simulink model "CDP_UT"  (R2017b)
settings: Solver=FixedStepDiscrete  StartTime=0.0  StopTime=10.0  FixedStep=0.01  RelTol=1e-3  EnableMultiTasking=on
undefined symbols (not defined in the file): ASWTYPE_FALSE, ASWTYPE_TRUE, CaCDP_CellTempNTCVoltTable_mV, CaCDP_CellTempTable_C, CaCDP_CMUPCBTempNTCVoltTable_mV, CaCDP_CMUPCBTempTable_C, CbCDP_DiffBusbarTempStateCheck_flg, CbCDP_DiffCellTempStateCheck_flg, CbCDP_DiffCellVoltStateCheck_flg, CbCDP_IgnorUpdateVld_flg, CbCDP_MaxBusbarTempStateCheck_flg, CbCDP_MaxCellTempStateCheck_flg, CbCDP_MaxCellVoltStateCheck_flg, CbCDP_MinBusbarTempStateCheck_flg, CbCDP_MinCellTempStateCheck_flg, CbCDP_MinCellVoltStateCheck_flg, CcCDP_AFETempConfig_numb, CcCDP_AFETempFltThd_C, CcCDP_AFETempFltThdHys_C, CcCDP_BusbarTempRngFltHiThrd_C, CcCDP_BusbarTempRngFltLowThrd_C, CcCDP_CellDiffFltLevel1_mV, CcCDP_CellDiffFltLevel2_mV, CcCDP_CellDiffFltLevel3_mV, CcCDP_CellTempLowerLimit_C, CcCDP_CellTempRngFltHiThrd_C, CcCDP_CellTempRngFltLowThrd_C, CcCDP_CellTempUpperLimit_C, CcCDP_CellVoltConfig_numb, CcCDP_CellVoltLowerLimit_mV, CcCDP_CellVoltRngHiThrd_mV, CcCDP_CellVoltRngLowThrd_mV, CcCDP_CellVoltUpdateThrd_numb, CcCDP_CellVoltUpperLimit_mV, CcCDP_ChrgMaxCellTempFltLv1Thrd_C, CcCDP_ChrgMaxCellTempFltLv2Thrd_C, CcCDP_ChrgMaxCellTempFltLv3Thrd_C, CcCDP_ChrgMaxCellTempReturnDiff_C, CcCDP_ChrgMinCellTempFltLv1Thrd_C, CcCDP_ChrgMinCellTempFltLv2Thrd_C, CcCDP_ChrgMinCellTempFltLv3Thrd_C, CcCDP_ChrgMinCellTempReturnDiff_C, CcCDP_CMUPCBTempConfig_numb, CcCDP_CMUPCBTempFltThd_C, CcCDP_CMUPCBTempFltThdHys_C, CcCDP_DiffBusbarTempFltLevel1Thrd_C, CcCDP_DiffBusbarTempFltLevel2Thrd_C, CcCDP_DiffBusbarTempReturnDifference_C, CcCDP_DiffCellTempFltLevel1Thrd_C, CcCDP_DiffCellTempFltLevel2Thrd_C, CcCDP_DiffCellTempReturnDifference_C, CcCDP_DiffCellVoltReturnDifference_mV, CcCDP_DiffVoltCheckMaxCellTempCondition_C, CcCDP_DiffVoltCheckMaxCellVoltCondition_mV, CcCDP_DiffVoltCheckMinCellTempCondition_C, CcCDP_DiffVoltCheckMinCellVoltCondition_mV, CcCDP_DiffVoltCheckPackCurrCondition_A, CcCDP_MaxAFETempIniVal_C, CcCDP_MaxBusbarTempFltLevel1Thrd_C, CcCDP_MaxBusbarTempFltLevel2Thrd_C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
libraries: AIWAYS_Powertrain_BMS_lib x148, simulink x8
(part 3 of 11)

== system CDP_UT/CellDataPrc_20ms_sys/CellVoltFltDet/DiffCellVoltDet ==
  LbCDP_CellVoltRngLowFlt_flg : Inport
  LbCDP_CellVoltRngHiFlt_flg : Inport  Port=2
  GcCDP_MinCellTemp_C : Inport  Port=3
  GcCDP_MaxCellVolt_mV : Inport  Port=4
  GcCDP_MinCellVolt_mV : Inport  Port=5
  LbCDP_AnyCellVoltVld_flg : Inport  Port=6
  GcCDP_MaxCellTemp_C : Inport  Port=7
  GcHDP_PackCrnt_A : Inport  Port=8
  GbHDP_PackCrntVld_flg : Inport  Port=9
  Bus Creator : BusCreator  Inputs=4
  Bus Selector : BusSelector  OutputSignals=GcCDP_MaxCellVolt_mV,GcCDP_MinCellVolt_mV,LbCDP_CellVoltRngLowFlt_flg,LbCDP_CellVoltRngHiFlt_flg
  Bus Selector1 : BusSelector  OutputSignals=GcCDP_MaxCellVolt_mV,GcCDP_MinCellVolt_mV
  DiffCellVolt_SateSwitch_Sys : Subsystem
  DiffVoltCheck_Condition : Subsystem
  GbCDP_CellVoltDiffFltLv3_flg : Outport
  GbCDP_CellVoltDiffFltLv2_flg : Outport  Port=2
  GbCDP_CellVoltDiffFltLv1_flg : Outport  Port=3
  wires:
  DiffVoltCheck_Condition/1(LbCDP_DiffvoltCheckCondition_flg) -> DiffCellVolt_SateSwitch_Sys/1(LbCDP_DiffvoltCheckCondition_flg)
  Bus Selector1/2 -> DiffVoltCheck_Condition/7(GcCDP_MinCellVolt_mV)  "<GcCDP_MinCellVolt_mV>"
  Bus Selector1/1 -> DiffVoltCheck_Condition/6(GcCDP_MaxCellVolt_mV)  "<GcCDP_MaxCellVolt_mV>"
  Bus Creator/1 -> Bus Selector/1, Bus Selector1/1
  GcCDP_MinCellVolt_mV/1 -> Bus Creator/2
  GcCDP_MaxCellVolt_mV/1 -> Bus Creator/1
  GcCDP_MinCellTemp_C/1 -> DiffVoltCheck_Condition/1(GcCDP_MinCellTemp_C)
  GbHDP_PackCrntVld_flg/1 -> DiffVoltCheck_Condition/5(GbHDP_PackCrntVld_flg)
  GcHDP_PackCrnt_A/1 -> DiffVoltCheck_Condition/4(GcHDP_PackCrnt_A)
  GcCDP_MaxCellTemp_C/1 -> DiffVoltCheck_Condition/3(GcCDP_MaxCellTemp_C)
  LbCDP_AnyCellVoltVld_flg/1 -> DiffVoltCheck_Condition/2(LbCDP_AnyCellVoltVld_flg)
  DiffCellVolt_SateSwitch_Sys/1(GbCDP_CellVoltDiffFltLv3_flg) -> GbCDP_CellVoltDiffFltLv3_flg/1
  DiffCellVolt_SateSwitch_Sys/2(GbCDP_CellVoltDiffFltLv2_flg) -> GbCDP_CellVoltDiffFltLv2_flg/1
  DiffCellVolt_SateSwitch_Sys/3(GbCDP_CellVoltDiffFltLv1_flg) -> GbCDP_CellVoltDiffFltLv1_flg/1
  LbCDP_CellVoltRngLowFlt_flg/1 -> Bus Creator/3
  LbCDP_CellVoltRngHiFlt_flg/1 -> Bus Creator/4
  Bus Selector/1 -> DiffCellVolt_SateSwitch_Sys/2(GcCDP_MaxCellVolt_mV)  "<GcCDP_MaxCellVolt_mV>"
  Bus Selector/2 -> DiffCellVolt_SateSwitch_Sys/3(GcCDP_MinCellVolt_mV)  "<GcCDP_MinCellVolt_mV>"
  Bus Selector/3 -> DiffCellVolt_SateSwitch_Sys/4(LbCDP_CellVoltRngLowFlt_flg)  "<LbCDP_CellVoltRngLowFlt_flg>"
  Bus Selector/4 -> DiffCellVolt_SateSwitch_Sys/5(LbCDP_CellVoltRngHiFlt_flg)  "<LbCDP_CellVoltRngHiFlt_flg>"

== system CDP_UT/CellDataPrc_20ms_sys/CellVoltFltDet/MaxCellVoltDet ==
  GbCDP_SumCellVoltVld_flg : Inport
  LcCDP_CellHighFltLevel1_mV : Inport  Port=2
  LcCDP_CellHighFltLevel2_mV : Inport  Port=3
  LcCDP_CellHighFltLevel3_mV : Inport  Port=4
  GcCDP_MaxCellVolt_mV : Inport  Port=5
  GeMSM_BMUState_enum : Inport  Port=6
  GbCTC_ChrgHVMode_flg : Inport  Port=7
  LbCDP_AnyCellVoltVld_flg : Inport  Port=8
  CellVoltHiFltDet : Subsystem
  MaxVoltCheck_Condition : Subsystem
  GbCDP_CellVoltHiFltLv3_flg : Outport
  GbCDP_CellVoltHiFltLv2_flg : Outport  Port=2
  GbCDP_CellVoltHiFltLv1_flg : Outport  Port=3
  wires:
  LcCDP_CellHighFltLevel3_mV/1 -> CellVoltHiFltDet/5(LcCDP_CellHighFltLevel3_mV)
  LcCDP_CellHighFltLevel2_mV/1 -> CellVoltHiFltDet/4(LcCDP_CellHighFltLevel2_mV)
  LcCDP_CellHighFltLevel1_mV/1 -> CellVoltHiFltDet/3(LcCDP_CellHighFltLevel1_mV)
  GcCDP_MaxCellVolt_mV/1 -> CellVoltHiFltDet/2(GcCDP_MaxCellVolt_mV)
  GbCDP_SumCellVoltVld_flg/1 -> MaxVoltCheck_Condition/1(GbCDP_SumCellVoltVld_flg)
  GeMSM_BMUState_enum/1 -> MaxVoltCheck_Condition/2(GeMSM_BMUState_enum)
  GbCTC_ChrgHVMode_flg/1 -> CellVoltHiFltDet/6(GbCTC_ChrgHVMode_flg)
  MaxVoltCheck_Condition/1(LbCDP_MaxVoltCheckCondition_flg) -> CellVoltHiFltDet/1(LbCDP_MaxVoltCheckCondition_flg)
  CellVoltHiFltDet/1(GbCDP_CellVoltHiFltLv3_flg) -> GbCDP_CellVoltHiFltLv3_flg/1
  CellVoltHiFltDet/2(GbCDP_CellVoltHiFltLv2_flg) -> GbCDP_CellVoltHiFltLv2_flg/1
  CellVoltHiFltDet/3(GbCDP_CellVoltHiFltLv1_flg) -> GbCDP_CellVoltHiFltLv1_flg/1
  LbCDP_AnyCellVoltVld_flg/1 -> MaxVoltCheck_Condition/3(LbCDP_AnyCellVoltVld_flg)

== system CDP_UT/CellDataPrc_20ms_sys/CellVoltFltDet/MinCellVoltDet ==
  GcCDP_MinCellVolt_mV : Inport
  LcCDP_CellLowFltLevel1_mV : Inport  Port=2
  LcCDP_CellLowFltLevel2_mV : Inport  Port=3
  LcCDP_CellLowFltLevel3_mV : Inport  Port=4
  GbCDP_SumCellVoltVld_flg : Inport  Port=5
  GeMSM_BMUState_enum : Inport  Port=6
  GbCTC_ChrgHVMode_flg : Inport  Port=7
  LbCDP_AnyCellVoltVld_flg : Inport  Port=8
  CellVoltLowFltDet : Subsystem
  MinVoltCheck_Condition : Subsystem
  GbCDP_CellVoltLowFltLv3_flg : Outport
  GbCDP_CellVoltLowFltLv2_flg : Outport  Port=2
  GbCDP_CellVoltLowFltLv1_flg : Outport  Port=3
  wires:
  LcCDP_CellLowFltLevel3_mV/1 -> CellVoltLowFltDet/5(LcCDP_CellLowFltLevel3_mV)
  LcCDP_CellLowFltLevel2_mV/1 -> CellVoltLowFltDet/4(LcCDP_CellLowFltLevel2_mV)
  LcCDP_CellLowFltLevel1_mV/1 -> CellVoltLowFltDet/3(LcCDP_CellLowFltLevel1_mV)
  GcCDP_MinCellVolt_mV/1 -> CellVoltLowFltDet/2(GcCDP_MinCellVolt_mV)
  GbCDP_SumCellVoltVld_flg/1 -> MinVoltCheck_Condition/1(GbCDP_SumCellVoltVld_flg)
  GeMSM_BMUState_enum/1 -> MinVoltCheck_Condition/2(GeMSM_BMUState_enum)
  GbCTC_ChrgHVMode_flg/1 -> CellVoltLowFltDet/6(GbCTC_ChrgHVMode_flg)
  CellVoltLowFltDet/2(GbCDP_CellVoltLowFltLv2_flg) -> GbCDP_CellVoltLowFltLv2_flg/1
  CellVoltLowFltDet/1(GbCDP_CellVoltLowFltLv3_flg) -> GbCDP_CellVoltLowFltLv3_flg/1
  CellVoltLowFltDet/3(GbCDP_CellVoltLowFltLv1_flg) -> GbCDP_CellVoltLowFltLv1_flg/1
  MinVoltCheck_Condition/1(LbCDP_MinVoltCheckCondition_flg) -> CellVoltLowFltDet/1(LbCDP_MinVoltCheckCondition_flg)
  LbCDP_AnyCellVoltVld_flg/1 -> MinVoltCheck_Condition/3(LbCDP_AnyCellVoltVld_flg)

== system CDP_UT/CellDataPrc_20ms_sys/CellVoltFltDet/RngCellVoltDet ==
  GcCDP_MinCellVolt_mV : Inport
  GeMSM_BMUState_enum : Inport  Port=2
  GcCDP_MaxCellVolt_mV : Inport  Port=3
  GbCDP_SumCellVoltVld_flg : Inport  Port=4
  LbCDP_AnyCellVoltVld_flg : Inport  Port=5
  Bus Creator : BusCreator  Inputs=3
  Bus Selector : BusSelector  OutputSignals=GbCDP_SumCellVoltVld_flg,GeMSM_BMUState_enum,LbCDP_AnyCellVoltVld_flg
  Bus Selector1 : BusSelector  OutputSignals=GbCDP_SumCellVoltVld_flg,GeMSM_BMUState_enum,LbCDP_AnyCellVoltVld_flg
  CellVoltRngHiCheck_Condition : Subsystem
  CellVoltRngHiFltDet : Subsystem
  CellVoltRngLowCheck_Condition : Subsystem
  CellVoltRngLowFltDet : Subsystem
  GbCDP_CellVoltRngLowFlt_flg : Outport
  GbCDP_CellVoltRngHiFlt_flg : Outport  Port=2
  LbCDP_CellVoltRngLowFlt_flg : Outport  Port=3
  LbCDP_CellVoltRngHiFlt_flg : Outport  Port=4
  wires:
  GeMSM_BMUState_enum/1 -> Bus Creator/2
  GcCDP_MinCellVolt_mV/1 -> CellVoltRngLowFltDet/2(GcCDP_MinCellVolt_mV)
  GbCDP_SumCellVoltVld_flg/1 -> Bus Creator/1
  CellVoltRngLowFltDet/1(GbCDP_CellVoltRngLowFlt_flg) -> GbCDP_CellVoltRngLowFlt_flg/1
  Bus Creator/1 -> Bus Selector1/1, Bus Selector/1
  Bus Selector/1 -> CellVoltRngLowCheck_Condition/1(GbCDP_SumCellVoltVld_flg)  "<GbCDP_SumCellVoltVld_flg>"
  Bus Selector/2 -> CellVoltRngLowCheck_Condition/2(GeMSM_BMUState_enum)  "<GeMSM_BMUState_enum>"
  Bus Selector1/1 -> CellVoltRngHiCheck_Condition/1(GbCDP_SumCellVoltVld_flg)  "<GbCDP_SumCellVoltVld_flg>"
  Bus Selector1/2 -> CellVoltRngHiCheck_Condition/2(GeMSM_BMUState_enum)  "<GeMSM_BMUState_enum>"
  GcCDP_MaxCellVolt_mV/1 -> CellVoltRngHiFltDet/2(GcCDP_MaxCellVolt_mV)
  CellVoltRngHiFltDet/1(GbCDP_CellVoltRngHiFlt_flg) -> GbCDP_CellVoltRngHiFlt_flg/1
  CellVoltRngLowCheck_Condition/1(LbCDP_CellVoltRngLowChk_flg) -> CellVoltRngLowFltDet/1(LbCDP_CellVoltRngLowChk_flg)
  CellVoltRngHiCheck_Condition/1(LbCDP_CellVoltRngHiChk_flg) -> CellVoltRngHiFltDet/1(LbCDP_CellVoltRngHiChk_flg)
  LbCDP_AnyCellVoltVld_flg/1 -> Bus Creator/3
  Bus Selector/3 -> CellVoltRngLowCheck_Condition/3(LbCDP_AnyCellVoltVld_flg)  "<LbCDP_AnyCellVoltVld_flg>"
  Bus Selector1/3 -> CellVoltRngHiCheck_Condition/3(LbCDP_AnyCellVoltVld_flg)  "<LbCDP_AnyCellVoltVld_flg>"
  CellVoltRngLowFltDet/2(LbCDP_CellVoltRngLowFlt_flg) -> LbCDP_CellVoltRngLowFlt_flg/1
  CellVoltRngHiFltDet/2(LbCDP_CellVoltRngHiFlt_flg) -> LbCDP_CellVoltRngHiFlt_flg/1

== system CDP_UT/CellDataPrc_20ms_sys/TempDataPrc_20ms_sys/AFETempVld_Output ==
  GeISP_CmuReIninSts_enum : Inport
  GaISP_AFETempVld_numb : Inport  Port=2
  Bitwise Logical Operator : simulink/Logic and Bit Operations/Bitwise Operator  logicop=AND  UseBitMask=on  BitMask=CDP_CONST7_NUMB  BitMaskRealWorld=Stored Integer
  CDP_GaCDP_CMUPCBTempVld_flg : AIWAYS_Powertrain_BMS_lib/Signals/OverWrite  OverWrite_Value=CaCDP_AFETempVldOvr_flg  OverWrite_flag=CbCDP_AFETempVldOvrSwt_flg
  Constant2 : Constant  Value=CDP_CONST7_NUMB
  Constant3 : Constant  Value=Enum_ISPCmuReIninSts.Enum_ISPCmuReIninSts_InintProcess
  Data Type Conversion : DataTypeConversion
  Logical Operator2 : Logic  Operator=OR  AllPortsSameDT=off  OutDataTypeStr=boolean
  Relational Operator1 : RelationalOperator  Operator===  OutDataTypeStr=boolean
  Relational Operator3 : RelationalOperator  Operator===  OutDataTypeStr=boolean
  GaCDP_AFETempVld_flg : Outport
  LaCDP_AFETempVld_flg : Outport  Port=2
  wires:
  GaISP_AFETempVld_numb/1 -> Bitwise Logical Operator/1
  CDP_GaCDP_CMUPCBTempVld_flg/1 -> GaCDP_AFETempVld_flg/1  "GaCDP_AFETempVld_flg"
  Logical Operator2/1 -> LaCDP_AFETempVld_flg/1, CDP_GaCDP_CMUPCBTempVld_flg/1  "LaCDP_AFETempVld_flg"
  Relational Operator3/1 -> Logical Operator2/1
  Constant2/1 -> Relational Operator3/1
  Data Type Conversion/1 -> Relational Operator1/1
  GeISP_CmuReIninSts_enum/1 -> Data Type Conversion/1
  Constant3/1 -> Relational Operator1/2
  Relational Operator1/1 -> Logical Operator2/2
  Bitwise Logical Operator/1 -> Relational Operator3/2

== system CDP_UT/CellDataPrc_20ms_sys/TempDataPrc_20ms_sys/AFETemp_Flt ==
  GcCDP_MaxAFETemp_C : Inport
  CDP_GbCDP_CMUTempHighFlt_flg : AIWAYS_Powertrain_BMS_lib/Signals/OverWrite  OverWrite_Value=CbCDP_AFETempHighFltOvr_flg  OverWrite_flag=CbCDP_AFETempHighFltOvrSwt_flg
  Constant1 : Constant  Value=CcCDP_AFETempFltThdHys_C
  Constant3 : Constant  Value=CcCDP_AFETempFltThd_C
  Hysteresis : AIWAYS_Powertrain_BMS_lib/Nonlinear Blocks/Hysteresis
  Sum1 : Sum  Inputs=-+  OutDataTypeStr=Inherit: Inherit via back propagation  RndMeth=Zero
  GbCDP_AFETempHighFlt_flg : Outport
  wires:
  Sum1/1 -> Hysteresis/1
  Constant1/1 -> Sum1/1
  Constant3/1 -> Sum1/2, Hysteresis/2
  GcCDP_MaxAFETemp_C/1 -> Hysteresis/3
  Hysteresis/1 -> CDP_GbCDP_CMUTempHighFlt_flg/1
  CDP_GbCDP_CMUTempHighFlt_flg/1 -> GbCDP_AFETempHighFlt_flg/1  "GbCDP_AFETempHighFlt_flg"

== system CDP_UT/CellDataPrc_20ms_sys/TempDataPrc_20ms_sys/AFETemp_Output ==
  GeISP_CmuReIninSts_enum : Inport
  GaISP_AFETemp_numb : Inport  Port=2
  GaISP_AFETempVld_numb : Inport  Port=3
  Bitwise Logical Operator : simulink/Logic and Bit Operations/Bitwise Operator  logicop=AND  UseBitMask=on  BitMask=CDP_CONST7_NUMB  BitMaskRealWorld=Stored Integer
  CDP_GaCDP_CMUPCBTemp_C : AIWAYS_Powertrain_BMS_lib/Signals/OverWrite  OverWrite_Value=CaCDP_AFETempOvr_C  OverWrite_flag=CbCDP_AFETempOvrSwt_flg
  Constant2 : Constant  Value=CDP_CONST7_NUMB
  Constant3 : Constant  Value=Enum_ISPCmuReIninSts.Enum_ISPCmuReIninSts_InintProcess
  Data Type Conversion : DataTypeConversion
  Data Type Conversion1 : DataTypeConversion
  Logical Operator2 : Logic  Operator=OR  AllPortsSameDT=off  OutDataTypeStr=boolean
  Relational Operator1 : RelationalOperator  Operator===  OutDataTypeStr=boolean
  Relational Operator2 : RelationalOperator  Operator=~=  OutDataTypeStr=boolean
  Switch : Switch  Criteria=u2 ~= 0
  Unit Delay : UnitDelay  SampleTime=-1  StateName=StateName
  GaCDP_AFETemp_C : Outport
  LaCDP_AFETemp_C : Outport  Port=2
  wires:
  GaISP_AFETempVld_numb/1 -> Bitwise Logical Operator/1
  CDP_GaCDP_CMUPCBTemp_C/1 -> GaCDP_AFETemp_C/1  "GaCDP_AFETemp_C"
  Data Type Conversion1/1 -> Switch/3
  Switch/1 -> Unit Delay/1, LaCDP_AFETemp_C/1, CDP_GaCDP_CMUPCBTemp_C/1  "LaCDP_AFETemp_C"
  GeISP_CmuReIninSts_enum/1 -> Data Type Conversion/1
  Logical Operator2/1 -> Switch/2
  Unit Delay/1 -> Switch/1
  Relational Operator1/1 -> Logical Operator2/2
  Constant3/1 -> Relational Operator1/2
  Data Type Conversion/1 -> Relational Operator1/1
  GaISP_AFETemp_numb/1 -> Data Type Conversion1/1
  Relational Operator2/1 -> Logical Operator2/1
  Constant2/1 -> Relational Operator2/2
  Bitwise Logical Operator/1 -> Relational Operator2/1

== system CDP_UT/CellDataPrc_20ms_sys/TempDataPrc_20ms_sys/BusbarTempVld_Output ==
  GeISP_CmuReIninSts_enum : Inport
  GaISP_BusbarTempVld_numb : Inport  Port=2
  Bitwise Logical Operator : simulink/Logic and Bit Operations/Bitwise Operator  logicop=AND  UseBitMask=on  BitMask=CDP_CONST97_NUMB  BitMaskRealWorld=Stored Integer
  Constant2 : Constant  Value=CDP_CONST0_NUMB
  Constant3 : Constant  Value=Enum_ISPCmuReIninSts.Enum_ISPCmuReIninSts_InintProcess
  Data Type Conversion : DataTypeConversion
  Logical Operator2 : Logic  Operator=OR  AllPortsSameDT=off  OutDataTypeStr=boolean
  OverWrite4 : AIWAYS_Powertrain_BMS_lib/Signals/OverWrite  OverWrite_Value=CaCDP_BusbarTempVldOvr_flg  OverWrite_flag=CbCDP_BusbarTempVldOvrSwt_flg
  Relational Operator1 : RelationalOperator  Operator===  OutDataTypeStr=boolean
  Relational Operator3 : RelationalOperator  Operator===  OutDataTypeStr=boolean
  LaCDP_BusbarTempVld_flg : Outport
  GaCDP_BusbarTempVld_flg : Outport  Port=2
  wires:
  Relational Operator1/1 -> Logical Operator2/2
  Constant3/1 -> Relational Operator1/2
  GeISP_CmuReIninSts_enum/1 -> Data Type Conversion/1
  Data Type Conversion/1 -> Relational Operator1/1
  Constant2/1 -> Relational Operator3/2
  Relational Operator3/1 -> Logical Operator2/1
  OverWrite4/1 -> GaCDP_BusbarTempVld_flg/1  "GaCDP_BusbarTempVld_flg"
  Logical Operator2/1 -> LaCDP_BusbarTempVld_flg/1, OverWrite4/1  "LaCDP_BusbarTempVld_flg"
  GaISP_BusbarTempVld_numb/1 -> Bitwise Logical Operator/1
  Bitwise Logical Operator/1 -> Relational Operator3/1

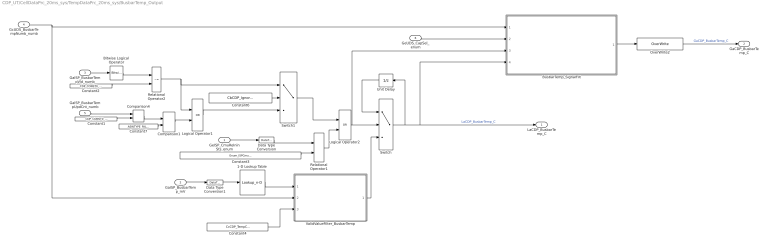
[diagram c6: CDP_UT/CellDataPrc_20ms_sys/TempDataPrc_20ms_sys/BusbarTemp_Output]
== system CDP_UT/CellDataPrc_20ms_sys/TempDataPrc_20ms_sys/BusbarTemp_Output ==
  GeISP_CmuReIninSts_enum : Inport
  GaISP_BusbarTemp_mV : Inport  Port=2
  GaISP_BusbarTempVld_numb : Inport  Port=3
  GcUDS_BusbarTempNumb_numb : Inport  Port=4
  GaISP_BusbarTempUpdCnt_numb : Inport  Port=5
  GeUDS_CapSel_enum : Inport  Port=6
  1-D Lookup Table : Lookup_n-D  NumberOfTableDimensions=1  BreakpointsForDimension1=CaCDP_CellTempNTCVoltTable_mV  Table=CaCDP_CellTempTable_C  ExtrapMethod=Clip  UseLastTableValue=on  InternalRulePriority=Speed  OutDataTypeStr=Inherit: Inherit from 'Table data'  RndMeth=Simplest
  Bitwise Logical Operator : simulink/Logic and Bit Operations/Bitwise Operator  logicop=AND  UseBitMask=on  BitMask=CDP_CONST97_NUMB  BitMaskRealWorld=Stored Integer
  BusbarTemp_SignalFilt : Subsystem
  Comparison1 : RelationalOperator  Operator===  OutDataTypeStr=boolean
  Comparison4 : RelationalOperator  Operator===  OutDataTypeStr=boolean
  Constant1 : Constant  Value=CDP_CONST0_NUMB
  Constant2 : Constant  Value=CDP_CONST0_NUMB
  Constant3 : Constant  Value=Enum_ISPCmuReIninSts.Enum_ISPCmuReIninSts_InintProcess
  Constant4 : Constant  Value=CcCDP_TempConfig_numb
  Constant6 : Constant  Value=CbCDP_IgnorUpdateVld_flg
  Constant7 : Constant  Value=ASWTYPE_FALSE
  Data Type Conversion : DataTypeConversion
  Data Type Conversion1 : DataTypeConversion
  Logical Operator1 : Logic  Operator=OR  AllPortsSameDT=off  OutDataTypeStr=boolean
  Logical Operator2 : Logic  Operator=OR  AllPortsSameDT=off  OutDataTypeStr=boolean
  OverWrite2 : AIWAYS_Powertrain_BMS_lib/Signals/OverWrite  OverWrite_Value=CaCDP_BusbarTempOvr_C  OverWrite_flag=CbCDP_BusbarTempOvrSwt_flg
  Relational Operator1 : RelationalOperator  Operator===  OutDataTypeStr=boolean
  Relational Operator2 : RelationalOperator  Operator=~=  OutDataTypeStr=boolean
  Switch : Switch  Criteria=u2 ~= 0
  Switch1 : Switch  Criteria=u2 ~= 0  Threshold=1  RndMeth=Zero
  Unit Delay : UnitDelay  SampleTime=-1  StateName=StateName
  ValidValueFilter_BusbarTemp : Stateflow chart  TreatAsAtomicUnit=on
  LaCDP_BusbarTemp_C : Outport
  GaCDP_BusbarTemp_C : Outport  Port=2
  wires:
  Constant2/1 -> Relational Operator2/2
  GaISP_BusbarTemp_mV/1 -> Data Type Conversion1/1
  Data Type Conversion/1 -> Relational Operator1/1
  Constant3/1 -> Relational Operator1/2
  Relational Operator1/1 -> Logical Operator2/2
  Unit Delay/1 -> Switch/1
  Logical Operator2/1 -> BusbarTemp_SignalFilt/3(LaCDP_BusbarTempUpdateVld_flg), Switch/2
  GeISP_CmuReIninSts_enum/1 -> Data Type Conversion/1
  Switch/1 -> BusbarTemp_SignalFilt/4(LaCDP_BusbarTemp_C), LaCDP_BusbarTemp_C/1, Unit Delay/1  "LaCDP_BusbarTemp_C"
  1-D Lookup Table/1 -> ValidValueFilter_BusbarTemp/1(InputValue)
  OverWrite2/1 -> GaCDP_BusbarTemp_C/1  "GaCDP_BusbarTemp_C"
  Data Type Conversion1/1 -> 1-D Lookup Table/1
  GaISP_BusbarTempVld_numb/1 -> Bitwise Logical Operator/1
  Bitwise Logical Operator/1 -> Relational Operator2/1
  GcUDS_BusbarTempNumb_numb/1 -> ValidValueFilter_BusbarTemp/2(NumbConfig), BusbarTemp_SignalFilt/1(GcUDS_BusbarTempNumb_numb)
  Constant4/1 -> ValidValueFilter_BusbarTemp/3(InputNumb)
  ValidValueFilter_BusbarTemp/1(OutputValue) -> Switch/3
  Constant6/1 -> Switch1/2
  Comparison4/1 -> Comparison1/1
  Relational Operator2/1 -> Switch1/1, Logical Operator1/1
  GaISP_BusbarTempUpdCnt_numb/1 -> Comparison4/1
  Constant7/1 -> Comparison1/2
  Comparison1/1 -> Logical Operator1/2
  Constant1/1 -> Comparison4/2
  Logical Operator1/1 -> Switch1/3
  Switch1/1 -> Logical Operator2/1
  BusbarTemp_SignalFilt/1(GaCDP_BusbarTemp_C) -> OverWrite2/1
  GeUDS_CapSel_enum/1 -> BusbarTemp_SignalFilt/2(GeUDS_CapSel_enum)

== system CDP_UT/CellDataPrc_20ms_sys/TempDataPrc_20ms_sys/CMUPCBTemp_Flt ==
  GcCDP_MaxCMUPCBTemp_C : Inport
  CDP_GbCDP_CMUTempHighFlt_flg : AIWAYS_Powertrain_BMS_lib/Signals/OverWrite  OverWrite_Value=CbCDP_CMUPCBTempHighFltOvr_flg  OverWrite_flag=CbCDP_CMUPCBTempHighFltOvrSwt_flg
  Constant1 : Constant  Value=CcCDP_CMUPCBTempFltThdHys_C
  Constant3 : Constant  Value=CcCDP_CMUPCBTempFltThd_C
  Hysteresis : AIWAYS_Powertrain_BMS_lib/Nonlinear Blocks/Hysteresis
  Sum1 : Sum  Inputs=-+  OutDataTypeStr=Inherit: Inherit via back propagation  RndMeth=Zero
  GbCDP_CMUPCBTempHighFlt_flg : Outport
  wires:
  CDP_GbCDP_CMUTempHighFlt_flg/1 -> GbCDP_CMUPCBTempHighFlt_flg/1  "GbCDP_CMUPCBTempHighFlt_flg"
  Hysteresis/1 -> CDP_GbCDP_CMUTempHighFlt_flg/1
  GcCDP_MaxCMUPCBTemp_C/1 -> Hysteresis/3
  Constant3/1 -> Hysteresis/2, Sum1/2
  Constant1/1 -> Sum1/1
  Sum1/1 -> Hysteresis/1

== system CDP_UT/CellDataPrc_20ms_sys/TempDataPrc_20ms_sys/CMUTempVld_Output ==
  GeISP_CmuReIninSts_enum : Inport
  GaISP_CMUPCBTempVld_numb : Inport  Port=2
  CDP_GaCDP_CMUPCBTempVld_flg : AIWAYS_Powertrain_BMS_lib/Signals/OverWrite  OverWrite_Value=CaCDP_CMUPCBTempVldOvr_flg  OverWrite_flag=CbCDP_CMUPCBTempVldOvrSwt_flg
  Constant2 : Constant  Value=CDP_CONST7_NUMB
  Constant3 : Constant  Value=Enum_ISPCmuReIninSts.Enum_ISPCmuReIninSts_InintProcess
  Data Type Conversion : DataTypeConversion
  Logical Operator2 : Logic  Operator=OR  AllPortsSameDT=off  OutDataTypeStr=boolean
  Relational Operator1 : RelationalOperator  Operator===  OutDataTypeStr=boolean
  Relational Operator3 : RelationalOperator  Operator===  OutDataTypeStr=boolean
  GaCDP_CMUPCBTempVld_flg : Outport
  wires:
  Relational Operator1/1 -> Logical Operator2/2
  Constant3/1 -> Relational Operator1/2
  GeISP_CmuReIninSts_enum/1 -> Data Type Conversion/1
  Data Type Conversion/1 -> Relational Operator1/1
  Constant2/1 -> Relational Operator3/1
  Relational Operator3/1 -> Logical Operator2/1
  Logical Operator2/1 -> CDP_GaCDP_CMUPCBTempVld_flg/1
  CDP_GaCDP_CMUPCBTempVld_flg/1 -> GaCDP_CMUPCBTempVld_flg/1  "GaCDP_CMUPCBTempVld_flg"
  GaISP_CMUPCBTempVld_numb/1 -> Relational Operator3/2

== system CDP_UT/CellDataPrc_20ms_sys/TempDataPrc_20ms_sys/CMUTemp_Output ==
  GeISP_CmuReIninSts_enum : Inport
  GaISP_CMUPCBTemp_mV : Inport  Port=2
  GaISP_CMUPCBTempVld_numb : Inport  Port=3
  1-D Lookup Table : Lookup_n-D  NumberOfTableDimensions=1  BreakpointsForDimension1=CaCDP_CMUPCBTempNTCVoltTable_mV  Table=CaCDP_CMUPCBTempTable_C  ExtrapMethod=Clip  UseLastTableValue=on  InternalRulePriority=Speed  OutDataTypeStr=Inherit: Inherit from 'Table data'  RndMeth=Simplest
  CDP_GaCDP_CMUPCBTemp_C : AIWAYS_Powertrain_BMS_lib/Signals/OverWrite  OverWrite_Value=CaCDP_CMUPCBTempOvr_C  OverWrite_flag=CbCDP_CMUPCBTempOvrSwt_flg
  Constant2 : Constant  Value=CDP_CONST7_NUMB
  Constant3 : Constant  Value=Enum_ISPCmuReIninSts.Enum_ISPCmuReIninSts_InintProcess
  Data Type Conversion : DataTypeConversion
  Data Type Conversion1 : DataTypeConversion
  Logical Operator2 : Logic  Operator=OR  AllPortsSameDT=off  OutDataTypeStr=boolean
  Relational Operator1 : RelationalOperator  Operator===  OutDataTypeStr=boolean
  Relational Operator2 : RelationalOperator  Operator=~=  OutDataTypeStr=boolean
  Switch : Switch  Criteria=u2 ~= 0
  Unit Delay : UnitDelay  SampleTime=-1  StateName=StateName
  GaCDP_CMUPCBTemp_C : Outport
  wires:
  Constant2/1 -> Relational Operator2/2
  Relational Operator2/1 -> Logical Operator2/1
  GaISP_CMUPCBTemp_mV/1 -> Data Type Conversion1/1
  Data Type Conversion/1 -> Relational Operator1/1
  Constant3/1 -> Relational Operator1/2
  Relational Operator1/1 -> Logical Operator2/2
  Unit Delay/1 -> Switch/1
  Logical Operator2/1 -> Switch/2
  GeISP_CmuReIninSts_enum/1 -> Data Type Conversion/1
  Switch/1 -> CDP_GaCDP_CMUPCBTemp_C/1, Unit Delay/1
  1-D Lookup Table/1 -> Switch/3
  Data Type Conversion1/1 -> 1-D Lookup Table/1
  CDP_GaCDP_CMUPCBTemp_C/1 -> GaCDP_CMUPCBTemp_C/1  "GaCDP_CMUPCBTemp_C"
  GaISP_CMUPCBTempVld_numb/1 -> Relational Operator2/1

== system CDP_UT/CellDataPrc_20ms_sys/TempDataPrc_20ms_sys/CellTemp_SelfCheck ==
  GeMSM_BMUState_enum : Inport
  GbCDP_AllCellTempVld_flg : Inport  Port=2
  GcCDP_MaxCellTemp_C : Inport  Port=3
  GcCDP_MinCellTemp_C : Inport  Port=4
  Constant : Constant  Value=Enum_MSMBMUState.Enum_MSMBMUState_Standby
  Constant1 : Constant  Value=ASWTYPE_TRUE
  Constant3 : Constant  Value=CcCDP_CellTempLowerLimit_C
  Constant4 : Constant  Value=CcCDP_CellTempUpperLimit_C
  Data Type Conversion1 : DataTypeConversion
  Logical Operator3 : Logic  Inputs=4  AllPortsSameDT=off  OutDataTypeStr=boolean
  OverWrite : AIWAYS_Powertrain_BMS_lib/Signals/OverWrite  OverWrite_Value=CbCDP_CellTempSelfChckOvr_flg  OverWrite_flag=CbCDP_CellTempSelfChckOvrSwt_flg
  Relational Operator : RelationalOperator  Operator===  OutDataTypeStr=boolean
  Relational Operator1 : RelationalOperator  Operator=<=  OutDataTypeStr=boolean
  Relational Operator3 : RelationalOperator  OutDataTypeStr=boolean
  Relational Operator4 : RelationalOperator  Operator===  OutDataTypeStr=boolean
  GbCDP_CellTempSelfChck_flg : Outport
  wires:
  GeMSM_BMUState_enum/1 -> Data Type Conversion1/1
  Constant/1 -> Relational Operator4/2
  Logical Operator3/1 -> OverWrite/1
  GcCDP_MinCellTemp_C/1 -> Relational Operator3/1
  Constant3/1 -> Relational Operator3/2
  Constant1/1 -> Relational Operator/2
  GbCDP_AllCellTempVld_flg/1 -> Relational Operator/1
  OverWrite/1 -> GbCDP_CellTempSelfChck_flg/1  "GbCDP_CellTempSelfChck_flg"
  GcCDP_MaxCellTemp_C/1 -> Relational Operator1/1
  Constant4/1 -> Relational Operator1/2
  Relational Operator4/1 -> Logical Operator3/1
  Relational Operator/1 -> Logical Operator3/2
  Relational Operator1/1 -> Logical Operator3/3
  Relational Operator3/1 -> Logical Operator3/4
  Data Type Conversion1/1 -> Relational Operator4/1

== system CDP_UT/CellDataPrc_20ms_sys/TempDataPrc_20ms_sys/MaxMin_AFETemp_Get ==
  LaCDP_AFETempVld_flg : Inport
  LaCDP_AFETemp_C : Inport  Port=2
  AllAFETemp_FaultCheck : Subsystem
  MaxMin_AFETemp_Get_Sys : Subsystem
  GcCDP_MaxAFETemp_C : Outport
  GcCDP_MinAFETemp_C : Outport  Port=2
  GcCDP_MaxAFETempNumb_numb : Outport  Port=3
  GcCDP_MinAFETempNumb_numb : Outport  Port=4
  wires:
  AllAFETemp_FaultCheck/1(LbCDP_AnyAFETempVld_flg) -> MaxMin_AFETemp_Get_Sys/Enable
  MaxMin_AFETemp_Get_Sys/4(GcCDP_MinAFETempNumb_numb) -> GcCDP_MinAFETempNumb_numb/1
  MaxMin_AFETemp_Get_Sys/3(GcCDP_MinAFETemp_C) -> GcCDP_MinAFETemp_C/1
  MaxMin_AFETemp_Get_Sys/2(GcCDP_MaxAFETempNumb_numb) -> GcCDP_MaxAFETempNumb_numb/1
  MaxMin_AFETemp_Get_Sys/1(GcCDP_MaxAFETemp_C) -> GcCDP_MaxAFETemp_C/1
  LaCDP_AFETemp_C/1 -> MaxMin_AFETemp_Get_Sys/2(LaCDP_AFETemp_C)
  LaCDP_AFETempVld_flg/1 -> AllAFETemp_FaultCheck/1(LaCDP_AFETempVld_flg), MaxMin_AFETemp_Get_Sys/1(LaCDP_AFETempVld_flg)

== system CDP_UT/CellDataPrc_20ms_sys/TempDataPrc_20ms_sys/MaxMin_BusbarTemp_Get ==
  GcUDS_BusbarTempNumb_numb : Inport
  LaCDP_BusbarTempVld_flg : Inport  Port=2
  LaCDP_BusbarTemp_C : Inport  Port=3
  GeUDS_CapSel_enum : Inport  Port=4
  GaISP_BusbarTempUpdCnt_numb : Inport  Port=5
  AllBusbarTemp_FaultCheck : Subsystem
  Bus Creator1 : BusCreator  Inputs=4
  Bus Selector1 : BusSelector  OutputSignals=LaCDP_BusbarTempVld_flg,GcUDS_BusbarTempNumb_numb,GaISP_BusbarTempUpdCnt_numb
  Bus Selector2 : BusSelector  OutputSignals=LaCDP_BusbarTempVld_flg,LaCDP_BusbarTemp_C,GcUDS_BusbarTempNumb_numb,GaISP_BusbarTempUpdCnt_numb
  Bus Selector3 : BusSelector  OutputSignals=LaCDP_BusbarTemp_C,GcUDS_BusbarTempNumb_numb
  BusbarTempMax_SignalFilt : Subsystem
  BusbarTempMin_SignalFilt : Subsystem
  MaxMin_BusbarAvgTemp_Get_Sys : Subsystem
  MaxMin_BusbarTemp_Get_Sys : Subsystem
  OverWrite : AIWAYS_Powertrain_BMS_lib/Signals/OverWrite  OverWrite_Value=CcCDP_MinBusbarTempOvr_C  OverWrite_flag=CbCDP_MinBusbarTempOvrSwt_flg
  OverWrite1 : AIWAYS_Powertrain_BMS_lib/Signals/OverWrite  OverWrite_Value=CcCDP_MinBusbarTempNumbOvr_numb  OverWrite_flag=CbCDP_MinBusbarTempNumbOvrSwt_flg
  OverWrite2 : AIWAYS_Powertrain_BMS_lib/Signals/OverWrite  OverWrite_Value=CcCDP_MaxBusbarTempOvr_C  OverWrite_flag=CbCDP_MaxBusbarTempOvrSwt_flg
  OverWrite3 : AIWAYS_Powertrain_BMS_lib/Signals/OverWrite  OverWrite_Value=CcCDP_MaxBusbarTempNumbOvr_numb  OverWrite_flag=CbCDP_MaxBusbarTempNumbOvrSwt_flg
  GbCDP_AllBusbarTempVld_flg : Outport
  GcCDP_MaxBusbarTemp_C : Outport  Port=2
  GcCDP_MinBusbarTemp_C : Outport  Port=3
  GcCDP_MaxBusbarTempNumb_numb : Outport  Port=4
  GcCDP_MinBusbarTempNumb_numb : Outport  Port=5
  GcCDP_AvgBusbarTemp_C : Outport  Port=6
  LbCDP_AnyBusbarTempVld_flg : Outport  Port=7
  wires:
  MaxMin_BusbarAvgTemp_Get_Sys/1(GcCDP_AvgBusbarTemp_C) -> GcCDP_AvgBusbarTemp_C/1
  AllBusbarTemp_FaultCheck/2(LbCDP_AnyBusbarTempVld_flg) -> LbCDP_AnyBusbarTempVld_flg/1, [LbCDP_AnyBusbarTempVld_flg], MaxMin_BusbarTemp_Get_Sys/Enable
  AllBusbarTemp_FaultCheck/1(GbCDP_AllBusbarTempVld_flg) -> GbCDP_AllBusbarTempVld_flg/1, MaxMin_BusbarAvgTemp_Get_Sys/Enable
  Bus Creator1/1 -> Bus Selector3/1, Bus Selector2/1, Bus Selector1/1
  GcUDS_BusbarTempNumb_numb/1 -> Bus Creator1/1
  LaCDP_BusbarTempVld_flg/1 -> Bus Creator1/2
  LaCDP_BusbarTemp_C/1 -> Bus Creator1/3
  Bus Selector1/1 -> AllBusbarTemp_FaultCheck/1(LaCDP_BusbarTempVld_flg)  "<LaCDP_BusbarTempVld_flg>"
  Bus Selector1/2 -> AllBusbarTemp_FaultCheck/2(GcUDS_BusbarTempNumb_numb)  "<GcUDS_BusbarTempNumb_numb>"
  Bus Selector2/1 -> MaxMin_BusbarTemp_Get_Sys/1(LaCDP_BusbarTempVld_flg)  "<LaCDP_BusbarTempVld_flg>"
  Bus Selector2/2 -> MaxMin_BusbarTemp_Get_Sys/2(LaCDP_BusbarTemp_C)  "<LaCDP_BusbarTemp_C>"
  Bus Selector2/3 -> MaxMin_BusbarTemp_Get_Sys/3(GcUDS_BusbarTempNumb_numb)  "<GcUDS_BusbarTempNumb_numb>"
  Bus Selector3/1 -> MaxMin_BusbarAvgTemp_Get_Sys/1(LaCDP_BusbarTemp_C)  "<LaCDP_BusbarTemp_C>"
  Bus Selector3/2 -> MaxMin_BusbarAvgTemp_Get_Sys/2(GcUDS_BusbarTempNumb_numb)  "<GcUDS_BusbarTempNumb_numb>"
  GaISP_BusbarTempUpdCnt_numb/1 -> Bus Creator1/4
  Bus Selector1/3 -> AllBusbarTemp_FaultCheck/3(GaISP_BusbarTempUpdCnt_numb)  "<GaISP_BusbarTempUpdCnt_numb>"
  OverWrite/1 -> GcCDP_MinBusbarTemp_C/1  "GcCDP_MinBusbarTemp_C"
  OverWrite1/1 -> GcCDP_MinBusbarTempNumb_numb/1  "GcCDP_MinBusbarTempNumb_numb"
  OverWrite3/1 -> GcCDP_MaxBusbarTempNumb_numb/1  "GcCDP_MaxBusbarTempNumb_numb"
  OverWrite2/1 -> GcCDP_MaxBusbarTemp_C/1  "GcCDP_MaxBusbarTemp_C"
  BusbarTempMax_SignalFilt/2(GcCDP_MaxBusbarTempNumb_numb) -> OverWrite3/1
  BusbarTempMax_SignalFilt/1(GcCDP_MaxBusbarTemp_C) -> OverWrite2/1
  BusbarTempMin_SignalFilt/2(GcCDP_MinBusbarTempNumb_numb) -> OverWrite1/1
  BusbarTempMin_SignalFilt/1(GcCDP_MinBusbarTemp_C) -> OverWrite/1
  MaxMin_BusbarTemp_Get_Sys/1(LcCDP_MaxBusbarTemp_C) -> BusbarTempMax_SignalFilt/1(LcCDP_MaxBusbarTemp_C)
  MaxMin_BusbarTemp_Get_Sys/2(LcCDP_MaxBusbarTempNumb_numb) -> BusbarTempMax_SignalFilt/2(LcCDP_MaxBusbarTempNumb_numb)
  [LbCDP_AnyBusbarTempVld_flg] -> BusbarTempMax_SignalFilt/3(LbCDP_AnyBusbarTempVld_flg)
  GeUDS_CapSel_enum/1 -> BusbarTempMin_SignalFilt/1(GeUDS_CapSel_enum), BusbarTempMax_SignalFilt/4(GeUDS_CapSel_enum)
  MaxMin_BusbarTemp_Get_Sys/3(LcCDP_MinBusbarTemp_C) -> BusbarTempMin_SignalFilt/3(LcCDP_MinBusbarTemp_C)
  MaxMin_BusbarTemp_Get_Sys/4(LcCDP_MinBusbarTempNumb_numb) -> BusbarTempMin_SignalFilt/4(LcCDP_MinBusbarTempNumb_numb)
  [LbCDP_AnyBusbarTempVld_flg] -> BusbarTempMin_SignalFilt/2(LbCDP_AnyBusbarTempVld_flg)
  Bus Selector2/4 -> MaxMin_BusbarTemp_Get_Sys/4(GaISP_BusbarTempUpdCnt_numb)  "<GaISP_BusbarTempUpdCnt_numb>"

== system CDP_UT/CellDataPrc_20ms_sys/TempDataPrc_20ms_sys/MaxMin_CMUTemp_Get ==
  GaCDP_CMUPCBTempVld_flg : Inport
  GaCDP_CMUPCBTemp_C : Inport  Port=2
  AllCMUPCBTemp_FaultCheck : Subsystem
  MaxMin_CMUPCBTemp_Get_Sys : Subsystem
  GcCDP_MaxCMUPCBTemp_C : Outport
  GcCDP_MinCMUPCBTemp_C : Outport  Port=2
  GcCDP_MaxCMUPCBTempNumb_numb : Outport  Port=3
  GcCDP_MinCMUPCBTempNumb_numb : Outport  Port=4
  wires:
  GaCDP_CMUPCBTempVld_flg/1 -> MaxMin_CMUPCBTemp_Get_Sys/1(GaCDP_CMUPCBTempVld_flg), AllCMUPCBTemp_FaultCheck/1(GaCDP_CMUPCBTempVld_flg)
  GaCDP_CMUPCBTemp_C/1 -> MaxMin_CMUPCBTemp_Get_Sys/2(GaCDP_CMUPCBTemp_C)
  MaxMin_CMUPCBTemp_Get_Sys/1(GcCDP_MaxCMUPCBTemp_C) -> GcCDP_MaxCMUPCBTemp_C/1
  MaxMin_CMUPCBTemp_Get_Sys/2(GcCDP_MaxCMUPCBTempNumb_numb) -> GcCDP_MaxCMUPCBTempNumb_numb/1
  MaxMin_CMUPCBTemp_Get_Sys/3(GcCDP_MinCMUPCBTemp_C) -> GcCDP_MinCMUPCBTemp_C/1
  MaxMin_CMUPCBTemp_Get_Sys/4(GcCDP_MinCMUPCBTempNumb_numb) -> GcCDP_MinCMUPCBTempNumb_numb/1
  AllCMUPCBTemp_FaultCheck/1(LbCDP_AnyCMUTempVld_flg) -> MaxMin_CMUPCBTemp_Get_Sys/Enable

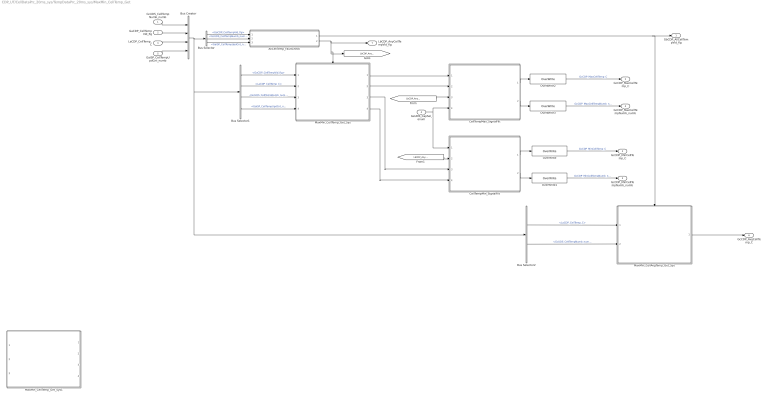
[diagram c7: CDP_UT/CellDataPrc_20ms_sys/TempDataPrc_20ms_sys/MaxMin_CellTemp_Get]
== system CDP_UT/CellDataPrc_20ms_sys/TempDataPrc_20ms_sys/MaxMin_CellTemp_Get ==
  GcUDS_CellTempNumb_numb : Inport
  GaCDP_CellTempVld_flg : Inport  Port=2
  LaCDP_CellTemp_C : Inport  Port=3
  GeUDS_CapSel_enum : Inport  Port=4
  GaISP_CellTempUpdCnt_numb : Inport  Port=5
  AllCellTemp_FaultCheck : Subsystem
  Bus Creator : BusCreator  Inputs=4
  Bus Selector : BusSelector  OutputSignals=GaCDP_CellTempVld_flg,GcUDS_CellTempNumb_numb,GaISP_CellTempUpdCnt_numb
  Bus Selector1 : BusSelector  OutputSignals=GaCDP_CellTempVld_flg,LaCDP_CellTemp_C,GcUDS_CellTempNumb_numb,GaISP_CellTempUpdCnt_numb
  Bus Selector2 : BusSelector  OutputSignals=LaCDP_CellTemp_C,GcUDS_CellTempNumb_numb
  CellTempMax_SignalFilt : Subsystem
  CellTempMin_SignalFilt : Subsystem
  MaxMin_CellAvgTemp_Get_Sys : Subsystem
  MaxMin_CellTemp_Get_Sys : Subsystem
  MaxMin_CellTemp_Get_Sys1 : Subsystem  Commented=on
  OverWrite : AIWAYS_Powertrain_BMS_lib/Signals/OverWrite  OverWrite_Value=CcCDP_MinCellTempOvr_C  OverWrite_flag=CbCDP_MinCellTempOvrSwt_flg
  OverWrite1 : AIWAYS_Powertrain_BMS_lib/Signals/OverWrite  OverWrite_Value=CcCDP_MinCellTempNumbOvr_numb  OverWrite_flag=CbCDP_MinCellTempNumbOvrSwt_flg
  OverWrite2 : AIWAYS_Powertrain_BMS_lib/Signals/OverWrite  OverWrite_Value=CcCDP_MaxCellTempOvr_C  OverWrite_flag=CbCDP_MaxCellTempOvrSwt_flg
  OverWrite3 : AIWAYS_Powertrain_BMS_lib/Signals/OverWrite  OverWrite_Value=CcCDP_MaxCellTempNumbOvr_numb  OverWrite_flag=CbCDP_MaxCellTempNumbOvrSwt_flg
  GbCDP_AllCellTempVld_flg : Outport
  GcCDP_MaxCellTemp_C : Outport  Port=2
  GcCDP_MinCellTemp_C : Outport  Port=3
  GcCDP_MaxCellTempNumb_numb : Outport  Port=4
  GcCDP_MinCellTempNumb_numb : Outport  Port=5
  GcCDP_AvgCellTemp_C : Outport  Port=6
  LbCDP_AnyCellTempVld_flg : Outport  Port=7
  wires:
  AllCellTemp_FaultCheck/1(GbCDP_AllCellTempVld_flg) -> GbCDP_AllCellTempVld_flg/1, MaxMin_CellAvgTemp_Get_Sys/Enable
  AllCellTemp_FaultCheck/2(LbCDP_AnyCellTempVld_flg) -> [LbCDP_AnyCellTempVld_flg], MaxMin_CellTemp_Get_Sys/Enable, LbCDP_AnyCellTempVld_flg/1
  MaxMin_CellAvgTemp_Get_Sys/1(GcCDP_AvgCellTemp_C) -> GcCDP_AvgCellTemp_C/1
  GcUDS_CellTempNumb_numb/1 -> Bus Creator/1
  GaCDP_CellTempVld_flg/1 -> Bus Creator/2
  LaCDP_CellTemp_C/1 -> Bus Creator/3
  Bus Creator/1 -> Bus Selector2/1, Bus Selector1/1, Bus Selector/1
  Bus Selector/1 -> AllCellTemp_FaultCheck/1(GaCDP_CellTempVld_flg)  "<GaCDP_CellTempVld_flg>"
  Bus Selector/2 -> AllCellTemp_FaultCheck/2(GcUDS_CellTempNumb_numb)  "<GcUDS_CellTempNumb_numb>"
  Bus Selector1/1 -> MaxMin_CellTemp_Get_Sys/1(GaCDP_CellTempVld_flg)  "<GaCDP_CellTempVld_flg>"
  Bus Selector1/2 -> MaxMin_CellTemp_Get_Sys/2(LaCDP_CellTemp_C)  "<LaCDP_CellTemp_C>"
  Bus Selector1/3 -> MaxMin_CellTemp_Get_Sys/3(GcUDS_CellTempNumb_numb)  "<GcUDS_CellTempNumb_numb>"
  Bus Selector2/1 -> MaxMin_CellAvgTemp_Get_Sys/1(LaCDP_CellTemp_C)  "<LaCDP_CellTemp_C>"
  Bus Selector2/2 -> MaxMin_CellAvgTemp_Get_Sys/2(GcUDS_CellTempNumb_numb)  "<GcUDS_CellTempNumb_numb>"
  MaxMin_CellTemp_Get_Sys/1(LcCDP_MaxCellTemp_C) -> CellTempMax_SignalFilt/1(LcCDP_MaxCellTemp_C)
  MaxMin_CellTemp_Get_Sys/2(LcCDP_MaxCellTempNumb_numb) -> CellTempMax_SignalFilt/2(LcCDP_MaxCellTempNumb_numb)
  [LbCDP_AnyCellTempVld_flg] -> CellTempMax_SignalFilt/3(LbCDP_AnyCellTempVld_flg)
  GeUDS_CapSel_enum/1 -> CellTempMin_SignalFilt/1(GeUDS_CapSel_enum), CellTempMax_SignalFilt/4(GeUDS_CapSel_enum)
  CellTempMax_SignalFilt/2(GcCDP_MaxCellTempNumb_numb) -> OverWrite3/1
  CellTempMin_SignalFilt/2(GcCDP_MinCellTempNumb_numb) -> OverWrite1/1
  CellTempMin_SignalFilt/1(GcCDP_MinCellTemp_C) -> OverWrite/1
  CellTempMax_SignalFilt/1(GcCDP_MaxCellTemp_C) -> OverWrite2/1
  OverWrite2/1 -> GcCDP_MaxCellTemp_C/1  "GcCDP_MaxCellTemp_C"
  OverWrite3/1 -> GcCDP_MaxCellTempNumb_numb/1  "GcCDP_MaxCellTempNumb_numb"
  OverWrite/1 -> GcCDP_MinCellTemp_C/1  "GcCDP_MinCellTemp_C"
  OverWrite1/1 -> GcCDP_MinCellTempNumb_numb/1  "GcCDP_MinCellTempNumb_numb"
  [LbCDP_AnyCellTempVld_flg] -> CellTempMin_SignalFilt/2(LbCDP_AnyCellTempVld_flg)
  MaxMin_CellTemp_Get_Sys/3(LcCDP_MinCellTemp_C) -> CellTempMin_SignalFilt/3(LcCDP_MinCellTemp_C)
  MaxMin_CellTemp_Get_Sys/4(LcCDP_MinCellTempNumb_numb) -> CellTempMin_SignalFilt/4(LcCDP_MinCellTempNumb_numb)
  GaISP_CellTempUpdCnt_numb/1 -> Bus Creator/4
  Bus Selector/3 -> AllCellTemp_FaultCheck/3(GaISP_CellTempUpdCnt_numb)  "<GaISP_CellTempUpdCnt_numb>"
  Bus Selector1/4 -> MaxMin_CellTemp_Get_Sys/4(GaISP_CellTempUpdCnt_numb)  "<GaISP_CellTempUpdCnt_numb>"

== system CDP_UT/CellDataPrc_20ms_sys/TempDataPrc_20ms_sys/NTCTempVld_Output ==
  GeISP_CmuReIninSts_enum : Inport
  GaISP_CellTempVld_numb : Inport  Port=2
  Bitwise Logical Operator : simulink/Logic and Bit Operations/Bitwise Operator  logicop=AND  UseBitMask=on  BitMask=CDP_CONST97_NUMB  BitMaskRealWorld=Stored Integer
  Constant2 : Constant  Value=CDP_CONST0_NUMB
  Constant3 : Constant  Value=Enum_ISPCmuReIninSts.Enum_ISPCmuReIninSts_InintProcess
  Data Type Conversion : DataTypeConversion
  Logical Operator2 : Logic  Operator=OR  AllPortsSameDT=off  OutDataTypeStr=boolean
  OverWrite4 : AIWAYS_Powertrain_BMS_lib/Signals/OverWrite  OverWrite_Value=CaCDP_CellTempVldOvr_flg  OverWrite_flag=CbCDP_CellTempVldOvrSwt_flg
  Relational Operator1 : RelationalOperator  Operator===  OutDataTypeStr=boolean
  Relational Operator3 : RelationalOperator  Operator===  OutDataTypeStr=boolean
  GaCDP_CellTempVld_flg : Outport
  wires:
  Relational Operator1/1 -> Logical Operator2/2
  Constant3/1 -> Relational Operator1/2
  GeISP_CmuReIninSts_enum/1 -> Data Type Conversion/1
  Data Type Conversion/1 -> Relational Operator1/1
  Constant2/1 -> Relational Operator3/2
  Relational Operator3/1 -> Logical Operator2/1
  OverWrite4/1 -> GaCDP_CellTempVld_flg/1  "GaCDP_CellTempVld_flg"
  Logical Operator2/1 -> OverWrite4/1
  GaISP_CellTempVld_numb/1 -> Bitwise Logical Operator/1
  Bitwise Logical Operator/1 -> Relational Operator3/1

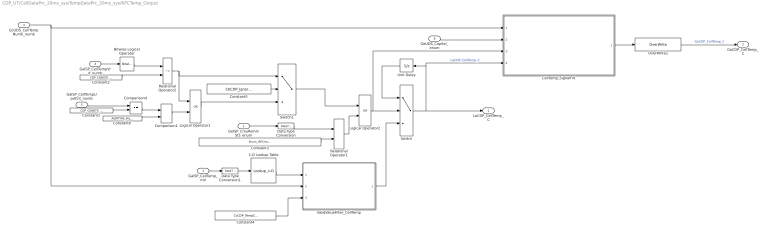
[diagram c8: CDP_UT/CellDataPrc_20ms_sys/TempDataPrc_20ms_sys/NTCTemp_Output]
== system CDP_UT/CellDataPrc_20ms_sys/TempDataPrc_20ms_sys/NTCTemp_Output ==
  GeISP_CmuReIninSts_enum : Inport
  GaISP_CellTemp_mV : Inport  Port=2
  GaISP_CellTempVld_numb : Inport  Port=3
  GcUDS_CellTempNumb_numb : Inport  Port=4
  GaISP_CellTempUpdCnt_numb : Inport  Port=5
  GeUDS_CapSel_enum : Inport  Port=6
  1-D Lookup Table : Lookup_n-D  NumberOfTableDimensions=1  BreakpointsForDimension1=CaCDP_CellTempNTCVoltTable_mV  Table=CaCDP_CellTempTable_C  ExtrapMethod=Clip  UseLastTableValue=on  InternalRulePriority=Speed  OutDataTypeStr=Inherit: Inherit from 'Table data'  RndMeth=Simplest
  Bitwise Logical Operator : simulink/Logic and Bit Operations/Bitwise Operator  logicop=AND  UseBitMask=on  BitMask=CDP_CONST97_NUMB  BitMaskRealWorld=Stored Integer
  CellTemp_SignalFilt : Subsystem
  Comparison1 : RelationalOperator  Operator===  OutDataTypeStr=boolean
  Comparison4 : RelationalOperator  Operator===  OutDataTypeStr=boolean
  Constant1 : Constant  Value=CDP_CONST0_NUMB
  Constant2 : Constant  Value=CDP_CONST0_NUMB
  Constant3 : Constant  Value=Enum_ISPCmuReIninSts.Enum_ISPCmuReIninSts_InintProcess
  Constant4 : Constant  Value=CcCDP_TempConfig_numb
  Constant5 : Constant  Value=CbCDP_IgnorUpdateVld_flg
  Constant6 : Constant  Value=ASWTYPE_FALSE
  Data Type Conversion : DataTypeConversion
  Data Type Conversion1 : DataTypeConversion
  Logical Operator1 : Logic  Operator=OR  AllPortsSameDT=off  OutDataTypeStr=boolean
  Logical Operator2 : Logic  Operator=OR  AllPortsSameDT=off  OutDataTypeStr=boolean
  OverWrite2 : AIWAYS_Powertrain_BMS_lib/Signals/OverWrite  OverWrite_Value=CaCDP_CellTempOvr_C  OverWrite_flag=CbCDP_CellTempOvrSwt_flg
  Relational Operator1 : RelationalOperator  Operator===  OutDataTypeStr=boolean
  Relational Operator2 : RelationalOperator  Operator=~=  OutDataTypeStr=boolean
  Switch : Switch  Criteria=u2 ~= 0
  Switch1 : Switch  Criteria=u2 ~= 0  Threshold=1  RndMeth=Zero
  Unit Delay : UnitDelay  SampleTime=-1  StateName=StateName
  ValidValueFilter_CellTemp : Stateflow chart  TreatAsAtomicUnit=on
  LaCDP_CellTemp_C : Outport
  GaCDP_CellTemp_C : Outport  Port=2
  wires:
  Constant2/1 -> Relational Operator2/2
  GaISP_CellTemp_mV/1 -> Data Type Conversion1/1
  Data Type Conversion/1 -> Relational Operator1/1
  Constant3/1 -> Relational Operator1/2
  Relational Operator1/1 -> Logical Operator2/2
  Unit Delay/1 -> Switch/1
  Logical Operator2/1 -> CellTemp_SignalFilt/3(LaCDP_CellTempUpdateVld_flg), Switch/2
  GeISP_CmuReIninSts_enum/1 -> Data Type Conversion/1
  Switch/1 -> LaCDP_CellTemp_C/1, CellTemp_SignalFilt/4(LaCDP_CellTemp_C), Unit Delay/1  "LaCDP_CellTemp_C"
  1-D Lookup Table/1 -> ValidValueFilter_CellTemp/1(InputValue)
  OverWrite2/1 -> GaCDP_CellTemp_C/1  "GaCDP_CellTemp_C"
  Data Type Conversion1/1 -> 1-D Lookup Table/1
  GaISP_CellTempVld_numb/1 -> Bitwise Logical Operator/1
  Bitwise Logical Operator/1 -> Relational Operator2/1
  GcUDS_CellTempNumb_numb/1 -> CellTemp_SignalFilt/1(GcUDS_CellTempNumb_numb), ValidValueFilter_CellTemp/2(NumbConfig)
  Constant4/1 -> ValidValueFilter_CellTemp/3(InputNumb)
  ValidValueFilter_CellTemp/1(OutputValue) -> Switch/3
  CellTemp_SignalFilt/1(GaCDP_CellTemp_C) -> OverWrite2/1
  Relational Operator2/1 -> Switch1/1, Logical Operator1/1
  Constant1/1 -> Comparison4/2
  Constant5/1 -> Switch1/2
  GaISP_CellTempUpdCnt_numb/1 -> Comparison4/1
  Logical Operator1/1 -> Switch1/3
  Comparison1/1 -> Logical Operator1/2
  Comparison4/1 -> Comparison1/1
  Constant6/1 -> Comparison1/2
  Switch1/1 -> Logical Operator2/1
  GeUDS_CapSel_enum/1 -> CellTemp_SignalFilt/2(GeUDS_CapSel_enum)

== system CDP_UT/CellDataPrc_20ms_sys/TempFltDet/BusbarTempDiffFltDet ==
  LbCDP_BusbarTempRngHiFlt_flg : Inport
  LbCDP_BusbarTempRngLowFlt_flg : Inport  Port=2
  LbCDP_AnyBusbarTempVld_flg : Inport  Port=3
  GcCDP_MaxBusbarTemp_C : Inport  Port=4
  GcCDP_MinBusbarTemp_C : Inport  Port=5
  BusbarTempDiffFltDet_Sys : Subsystem
  DiffTempCheck_Condition : Subsystem
  GbCDP_BusbarTempDiffFltLv2_flg : Outport
  GbCDP_BusbarTempDiffFltLv1_flg : Outport  Port=2
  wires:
  DiffTempCheck_Condition/1(LbCDP_DiffBusbarTempChkCond_flg) -> BusbarTempDiffFltDet_Sys/1(LbCDP_DiffBusbarTempChkCond_flg)
  BusbarTempDiffFltDet_Sys/2(GbCDP_BusbarTempDiffFltLv1_flg) -> GbCDP_BusbarTempDiffFltLv1_flg/1
  BusbarTempDiffFltDet_Sys/1(GbCDP_BusbarTempDiffFltLv2_flg) -> GbCDP_BusbarTempDiffFltLv2_flg/1
  LbCDP_BusbarTempRngLowFlt_flg/1 -> BusbarTempDiffFltDet_Sys/5(LbCDP_BusbarTempRngLowFlt_flg)
  LbCDP_BusbarTempRngHiFlt_flg/1 -> BusbarTempDiffFltDet_Sys/4(LbCDP_BusbarTempRngHiFlt_flg)
  LbCDP_AnyBusbarTempVld_flg/1 -> DiffTempCheck_Condition/1(LbCDP_AnyBusbarTempVld_flg)
  GcCDP_MinBusbarTemp_C/1 -> BusbarTempDiffFltDet_Sys/3(GcCDP_MinBusbarTemp_C)
  GcCDP_MaxBusbarTemp_C/1 -> BusbarTempDiffFltDet_Sys/2(GcCDP_MaxBusbarTemp_C)

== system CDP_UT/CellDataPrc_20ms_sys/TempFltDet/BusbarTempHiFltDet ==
  LbCDP_AnyBusbarTempVld_flg : Inport
  GcCDP_MaxBusbarTemp_C : Inport  Port=2
  BusbarTempHiFltDet_sys : Subsystem
  MaxBusbarTempCheck_Condition : Subsystem
  GbCDP_BusbarTempHiFltLv3_flg : Outport
  GbCDP_BusbarTempHiFltLv2_flg : Outport  Port=2
  GbCDP_BusbarTempHiFltLv1_flg : Outport  Port=3
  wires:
  GcCDP_MaxBusbarTemp_C/1 -> BusbarTempHiFltDet_sys/2(GcCDP_MaxBusbarTemp_C)
  LbCDP_AnyBusbarTempVld_flg/1 -> MaxBusbarTempCheck_Condition/1(LbCDP_AnyBusbarTempVld_flg)
  MaxBusbarTempCheck_Condition/1(LbCDP_MaxBusbarTempChkCond_flg) -> BusbarTempHiFltDet_sys/1(LbCDP_MaxBusbarTempChkCond_flg)
  BusbarTempHiFltDet_sys/1(GbCDP_BusbarTempHiFltLv3_flg) -> GbCDP_BusbarTempHiFltLv3_flg/1
  BusbarTempHiFltDet_sys/2(GbCDP_BusbarTempHiFltLv2_flg) -> GbCDP_BusbarTempHiFltLv2_flg/1
  BusbarTempHiFltDet_sys/3(GbCDP_BusbarTempHiFltLv1_flg) -> GbCDP_BusbarTempHiFltLv1_flg/1

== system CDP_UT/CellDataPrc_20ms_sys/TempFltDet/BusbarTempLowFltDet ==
  LbCDP_AnyBusbarTempVld_flg : Inport
  GcCDP_MinBusbarTemp_C : Inport  Port=2
  BusbarTempLowFltDet_sys : Subsystem
  MinBusbarTempCheck_Condition : Subsystem
  GbCDP_BusbarTempLowFltLv3_flg : Outport
  GbCDP_BusbarTempLowFltLv2_flg : Outport  Port=2
  GbCDP_BusbarTempLowFltLv1_flg : Outport  Port=3
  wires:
  GcCDP_MinBusbarTemp_C/1 -> BusbarTempLowFltDet_sys/2(GcCDP_MinBusbarTemp_C)
  LbCDP_AnyBusbarTempVld_flg/1 -> MinBusbarTempCheck_Condition/1(LbCDP_AnyBusbarTempVld_flg)
  MinBusbarTempCheck_Condition/1(LbCDP_MinBusbarTempChkCond_flg) -> BusbarTempLowFltDet_sys/1(LbCDP_MinBusbarTempChkCond_flg)
  BusbarTempLowFltDet_sys/1(GbCDP_BusbarTempLowFltLv3_flg) -> GbCDP_BusbarTempLowFltLv3_flg/1
  BusbarTempLowFltDet_sys/2(GbCDP_BusbarTempLowFltLv2_flg) -> GbCDP_BusbarTempLowFltLv2_flg/1
  BusbarTempLowFltDet_sys/3(GbCDP_BusbarTempLowFltLv1_flg) -> GbCDP_BusbarTempLowFltLv1_flg/1

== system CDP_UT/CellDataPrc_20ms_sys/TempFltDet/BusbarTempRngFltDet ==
  GcCDP_MaxBusbarTemp_C : Inport
  GcCDP_MinBusbarTemp_C : Inport  Port=2
  LbCDP_AnyBusbarTempVld_flg : Inport  Port=3
  BusbarTempRngHiFltDet_sys : Subsystem
  BusbarTempRngLowFltDet_sys : Subsystem
  TempRngHiCheck_Condition : Subsystem
  TempRngLowCheck_Condition : Subsystem
  GbCDP_BusbarTempRngHiFlt_flg : Outport
  GbCDP_BusbarTempRngLowFlt_flg : Outport  Port=2
  LbCDP_BusbarTempRngHiFlt_flg : Outport  Port=3
  LbCDP_BusbarTempRngLowFlt_flg : Outport  Port=4
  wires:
  TempRngHiCheck_Condition/1(LbCDP_BusbarTempRngHiChk_flg) -> BusbarTempRngHiFltDet_sys/1(LbCDP_BusbarTempRngHiChk_flg)
  BusbarTempRngLowFltDet_sys/2(GbCDP_BusbarTempRngLowFlt_flg) -> GbCDP_BusbarTempRngLowFlt_flg/1
  BusbarTempRngLowFltDet_sys/1(LbCDP_BusbarTempRngLowFlt_flg) -> LbCDP_BusbarTempRngLowFlt_flg/1
  TempRngLowCheck_Condition/1(LbCDP_BusbarTempRngLowChk_flg) -> BusbarTempRngLowFltDet_sys/1(LbCDP_BusbarTempRngLowChk_flg)
  GcCDP_MinBusbarTemp_C/1 -> BusbarTempRngLowFltDet_sys/2(GcCDP_MinBusbarTemp_C)
  BusbarTempRngHiFltDet_sys/2(GbCDP_BusbarTempRngHiFlt_flg) -> GbCDP_BusbarTempRngHiFlt_flg/1
  BusbarTempRngHiFltDet_sys/1(LbCDP_BusbarTempRngHiFlt_flg) -> LbCDP_BusbarTempRngHiFlt_flg/1
  LbCDP_AnyBusbarTempVld_flg/1 -> TempRngHiCheck_Condition/1(LbCDP_AnyBusbarTempVld_flg), TempRngLowCheck_Condition/1(LbCDP_AnyBusbarTempVld_flg)
  GcCDP_MaxBusbarTemp_C/1 -> BusbarTempRngHiFltDet_sys/2(GcCDP_MaxBusbarTemp_C)

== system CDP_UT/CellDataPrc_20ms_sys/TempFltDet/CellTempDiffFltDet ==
  LbCDP_CellTempRngHiFlt_flg : Inport
  LbCDP_CellTempRngLowFlt_flg : Inport  Port=2
  LbCDP_AnyCellTempVld_flg : Inport  Port=3
  GcCDP_MaxCellTemp_C : Inport  Port=4
  GcCDP_MinCellTemp_C : Inport  Port=5
  CellTempDiffFltDet_Sys : Subsystem
  DiffTempCheck_Condition : Subsystem
  GbCDP_CellTempDiffFltLv2_flg : Outport
  GbCDP_CellTempDiffFltLv1_flg : Outport  Port=2
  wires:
  GcCDP_MaxCellTemp_C/1 -> CellTempDiffFltDet_Sys/2(GcCDP_MaxCellTemp_C)
  GcCDP_MinCellTemp_C/1 -> CellTempDiffFltDet_Sys/3(GcCDP_MinCellTemp_C)
  LbCDP_AnyCellTempVld_flg/1 -> DiffTempCheck_Condition/1(LbCDP_AnyCellTempVld_flg)
  LbCDP_CellTempRngHiFlt_flg/1 -> CellTempDiffFltDet_Sys/4(LbCDP_CellTempRngHiFlt_flg)
  LbCDP_CellTempRngLowFlt_flg/1 -> CellTempDiffFltDet_Sys/5(LbCDP_CellTempRngLowFlt_flg)
  CellTempDiffFltDet_Sys/1(GbCDP_CellTempDiffFltLv2_flg) -> GbCDP_CellTempDiffFltLv2_flg/1
  CellTempDiffFltDet_Sys/2(GbCDP_CellTempDiffFltLv1_flg) -> GbCDP_CellTempDiffFltLv1_flg/1
  DiffTempCheck_Condition/1(LbCDP_DiffTempCheckCondition_flg) -> CellTempDiffFltDet_Sys/1(LbCDP_DiffTempCheckCondition_flg)

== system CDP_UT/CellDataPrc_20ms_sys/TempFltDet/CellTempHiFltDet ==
  GbCDP_AllCellTempVld_flg : Inport
  GcCDP_MaxCellTemp_C : Inport  Port=2
  LbCDP_AnyCellTempVld_flg : Inport  Port=3
  LbCDP_ChrgWkUp_flg : Inport  Port=4
  CellTempHiFltDet_sys : Subsystem
  MaxTempCheck_Condition : Subsystem
  GbCDP_CellTempHiFltLv3_flg : Outport
  GbCDP_CellTempHiFltLv2_flg : Outport  Port=2
  GbCDP_CellTempHiFltLv1_flg : Outport  Port=3
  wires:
  GcCDP_MaxCellTemp_C/1 -> CellTempHiFltDet_sys/2(GcCDP_MaxCellTemp_C)
  GbCDP_AllCellTempVld_flg/1 -> MaxTempCheck_Condition/1(GbCDP_AllCellTempVld_flg)
  CellTempHiFltDet_sys/1(GbCDP_CellTempHiFltLv3_flg) -> GbCDP_CellTempHiFltLv3_flg/1
  CellTempHiFltDet_sys/2(GbCDP_CellTempHiFltLv2_flg) -> GbCDP_CellTempHiFltLv2_flg/1
  CellTempHiFltDet_sys/3(GbCDP_CellTempHiFltLv1_flg) -> GbCDP_CellTempHiFltLv1_flg/1
  LbCDP_AnyCellTempVld_flg/1 -> MaxTempCheck_Condition/2(LbCDP_AnyCellTempVld_flg)
  MaxTempCheck_Condition/1(LbCDP_MaxTempCheckCondition_flg) -> CellTempHiFltDet_sys/1(LbCDP_MaxTempCheckCondition_flg)
  LbCDP_ChrgWkUp_flg/1 -> MaxTempCheck_Condition/3(LbCDP_ChrgWkUp_flg)
